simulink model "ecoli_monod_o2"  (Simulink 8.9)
settings: Solver=ode45  StartTime=6.69  StopTime=11.57  MaxStep=0.5  RelTol=1e-6  AbsTol=1e-6  EnableMultiTasking=on
undefined symbols (not defined in the file or in its folder): DO0, DOo, F, K1, k3, Kla, Ks, Mmax, S0, So, V, X0

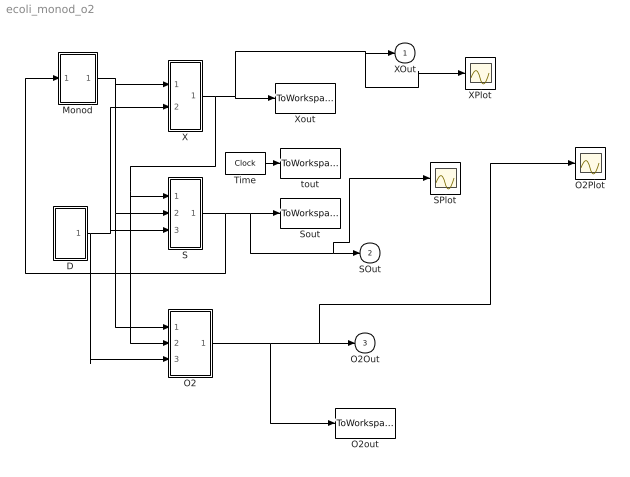
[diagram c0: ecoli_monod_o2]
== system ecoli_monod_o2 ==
  D : Subsystem
  Monod : Subsystem
  O2 : Subsystem
  O2Plot : Scope
  O2out : ToWorkspace  VariableName=O2out  SampleTime=-1
  S : Subsystem
  SPlot : Scope
  Sout : ToWorkspace  VariableName=Sout  SampleTime=-1
  Time : Clock
  X : Subsystem
  XPlot : Scope
  Xout : ToWorkspace  VariableName=Xout  SampleTime=-1
  tout : ToWorkspace  VariableName=tout  SampleTime=-1
  XOut : Outport
  SOut : Outport  Port=2
  O2Out : Outport  Port=3
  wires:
  S/1(Sout) -> Monod/1(S), Sout/1, SPlot/1, SOut/1
  Time/1 -> tout/1
  Monod/1(mu) -> X/1(mu), S/2(mu), O2/1(mu)
  D/1(out_1) -> S/3(F/V), X/2(F/V), O2/3(F/V)
  O2/1(DOout) -> O2out/1, O2Plot/1, O2Out/1
  X/1(XOut) -> Xout/1, XPlot/1, XOut/1, S/1(X), O2/2(X)

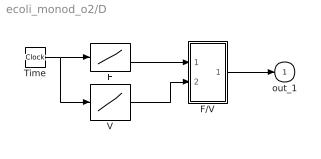
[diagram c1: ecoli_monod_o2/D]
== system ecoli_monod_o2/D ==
  F : Lookup  InputValues=t  Table=F
  F/V : Subsystem
  Time : Clock
  V : Lookup  InputValues=t  Table=V
  out_1 : Outport
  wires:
  F/V/1(out_1) -> out_1/1
  F/1 -> F/V/1(F)
  V/1 -> F/V/2(V)
  Time/1 -> F/1, V/1

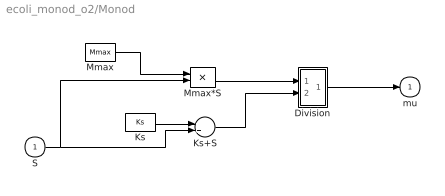
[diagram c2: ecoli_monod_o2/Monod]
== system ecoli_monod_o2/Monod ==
  S : Inport
  Division : Subsystem
  Ks : Constant  Value=Ks
  Ks+S : Sum
  Mmax : Constant  Value=Mmax
  Mmax*S : Product
  mu : Outport
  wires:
  Division/1(out_1) -> mu/1
  Mmax/1 -> Mmax*S/1
  Mmax*S/1 -> Division/1(Mmax*S)
  Ks+S/1 -> Division/2(Ks+S)
  Ks/1 -> Ks+S/1
  S/1 -> Ks+S/2, Mmax*S/2

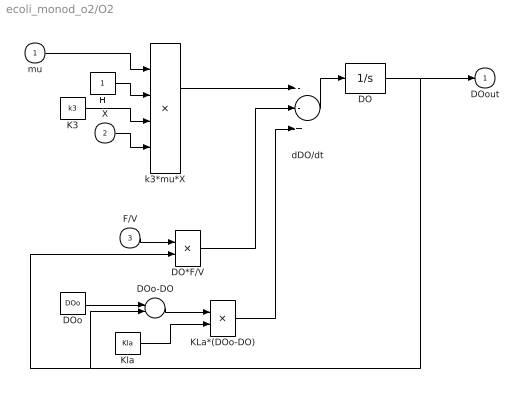
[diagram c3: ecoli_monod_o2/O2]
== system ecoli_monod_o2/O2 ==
  mu : Inport
  X : Inport  Port=2
  F/V : Inport  Port=3
  DO : Integrator  InitialCondition=DO0  UpperSaturationLimit=1000  LowerSaturationLimit=0
  DO*F/V : Product
  DOo : Constant  Value=DOo
  DOo-DO : Sum  Inputs=+-
  H : Constant
  K3 : Constant  Value=k3
  KLa*(DOo-DO) : Product
  Kla : Constant  Value=Kla
  dDO/dt : Sum  Inputs=--+
  k3*mu*X : Product  Inputs=4
  DOout : Outport
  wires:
  DO/1 -> DOout/1, DOo-DO/2, DO*F/V/2
  dDO/dt/1 -> DO/1
  k3*mu*X/1 -> dDO/dt/1
  DOo-DO/1 -> KLa*(DOo-DO)/1
  DOo/1 -> DOo-DO/1
  Kla/1 -> KLa*(DOo-DO)/2
  KLa*(DOo-DO)/1 -> dDO/dt/3
  F/V/1 -> DO*F/V/1
  DO*F/V/1 -> dDO/dt/2
  mu/1 -> k3*mu*X/1
  H/1 -> k3*mu*X/2
  K3/1 -> k3*mu*X/3
  X/1 -> k3*mu*X/4

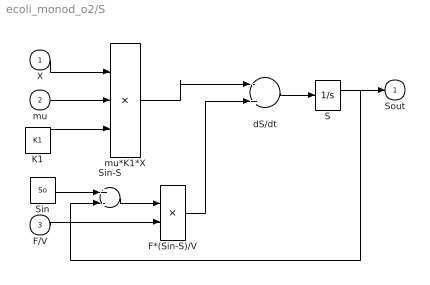
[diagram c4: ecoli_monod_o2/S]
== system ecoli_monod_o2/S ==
  X : Inport
  mu : Inport  Port=2
  F/V : Inport  Port=3
  F*(Sin-S)/V : Product
  K1 : Constant  Value=K1
  S : Integrator  InitialCondition=S0  UpperSaturationLimit=1000  LowerSaturationLimit=0
  Sin : Constant  Value=So
  Sin-S : Sum  Inputs=+-
  dS/dt : Sum  Inputs=-+
  mu*K1*X : Product  Inputs=3
  Sout : Outport
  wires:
  S/1 -> Sout/1, Sin-S/2
  Sin-S/1 -> F*(Sin-S)/V/1
  Sin/1 -> Sin-S/1
  X/1 -> mu*K1*X/1
  F/V/1 -> F*(Sin-S)/V/2
  mu*K1*X/1 -> dS/dt/1
  F*(Sin-S)/V/1 -> dS/dt/2
  dS/dt/1 -> S/1
  mu/1 -> mu*K1*X/2
  K1/1 -> mu*K1*X/3

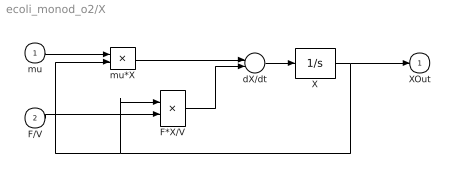
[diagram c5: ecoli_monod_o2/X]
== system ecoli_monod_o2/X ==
  mu : Inport
  F/V : Inport  Port=2
  F*X/V : Product
  X : Integrator  InitialCondition=X0  UpperSaturationLimit=1000  LowerSaturationLimit=0
  dX/dt : Sum  Inputs=+-
  mu*X : Product
  XOut : Outport
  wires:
  F*X/V/1 -> dX/dt/2
  dX/dt/1 -> X/1
  mu*X/1 -> dX/dt/1
  mu/1 -> mu*X/1
  X/1 -> XOut/1, mu*X/2, F*X/V/1
  F/V/1 -> F*X/V/2

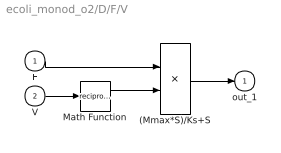
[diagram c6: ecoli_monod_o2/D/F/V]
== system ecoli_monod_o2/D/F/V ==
  F : Inport
  V : Inport  Port=2
  (Mmax*S)/Ks+S : Product
  Math Function : Math  Operator=reciprocal
  out_1 : Outport
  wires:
  F/1 -> (Mmax*S)/Ks+S/1
  V/1 -> Math Function/1
  Math Function/1 -> (Mmax*S)/Ks+S/2
  (Mmax*S)/Ks+S/1 -> out_1/1

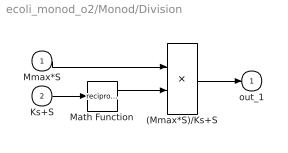
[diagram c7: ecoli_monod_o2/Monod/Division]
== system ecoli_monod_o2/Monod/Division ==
  Mmax*S : Inport
  Ks+S : Inport  Port=2
  (Mmax*S)/Ks+S : Product
  Math Function : Math  Operator=reciprocal
  out_1 : Outport
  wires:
  Mmax*S/1 -> (Mmax*S)/Ks+S/1
  Ks+S/1 -> Math Function/1
  Math Function/1 -> (Mmax*S)/Ks+S/2
  (Mmax*S)/Ks+S/1 -> out_1/1
